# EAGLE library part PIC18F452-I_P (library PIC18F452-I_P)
Microcontroller,PIC18F452-I/P 40MHz Microchip PIC18F452-I/P, 8bit PIC Microcontroller, 40MHz, 32 kB Flash, 40-Pin PDIP Source: Datasheet
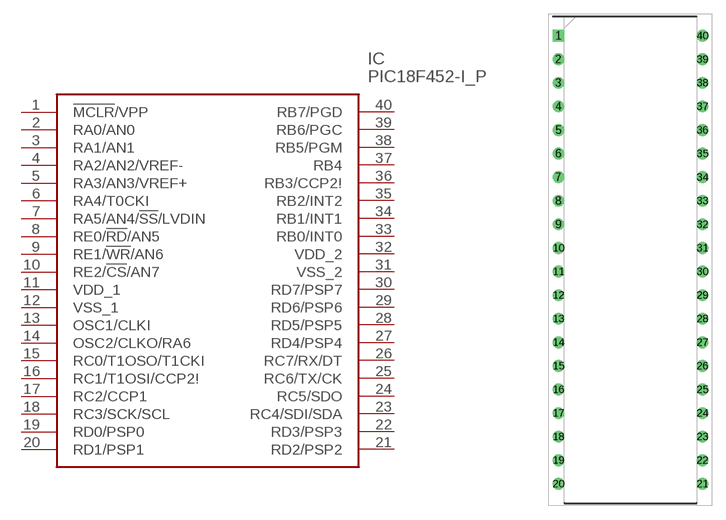
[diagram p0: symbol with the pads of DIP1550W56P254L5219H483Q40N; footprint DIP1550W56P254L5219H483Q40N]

Designator prefix IC

## PIC18F452-I_P (Description: Microcontroller,PIC18F452-I/P 40MHz Microchip PIC18F452-I/P, 8bit PIC Microcontroller, 40MHz, 32 kB Flash, 40-Pin PDIP; Height: 4.83mm; Manufacturer_Name: Microchip; Manufacturer_Part_Number: PIC18F452-I/P; Mouser_Part_Number: 579-PIC18F452-I/P; Mouser_Price-Stock: https://www.mouser.co.uk/ProductDetail/Microchip-Technology-Atmel/PIC18F452-I-P?qs=huzeVNXgovVccIn1hiWGAA%3D%3D)  [DIP1550W56P254L5219H483Q40N]
1  !MCLR!/VPP
2  RA0/AN0
3  RA1/AN1
4  RA2/AN2/VREF-  in
5  RA3/AN3/VREF+  in
6  RA4/T0CKI
7  RA5/AN4/!SS!/LVDIN  in
8  RE0/!RD!/AN5
9  RE1/!WR!/AN6
10  RE2/!CS!/AN7  in
11  VDD_1  pwr
12  VSS_1  pwr
13  OSC1/CLKI  in
14  OSC2/CLKO/RA6  out
15  RC0/T1OSO/T1CKI
16  RC1/T1OSI/CCP2!
17  RC2/CCP1
18  RC3/SCK/SCL
19  RD0/PSP0
20  RD1/PSP1
21  RD2/PSP2
22  RD3/PSP3
23  RC4/SDI/SDA
24  RC5/SDO
25  RC6/TX/CK
26  RC7/RX/DT
27  RD4/PSP4
28  RD5/PSP5
29  RD6/PSP6
30  RD7/PSP7
31  VSS_2  pwr
32  VDD_2  pwr
33  RB0/INT0  in
34  RB1/INT1  in
35  RB2/INT2  in
36  RB3/CCP2!
37  RB4
38  RB5/PGM
39  RB6/PGC
40  RB7/PGD

## Footprint DIP1550W56P254L5219H483Q40N (pad centres in mm)
40-Lead Plastic Dual In-Line (P) - 600 mil Body [PDIP]
drill 0.76 pad 1.16 square: 1 -7.748,24.13
drill 0.76 pad 1.16: 2 -7.748,21.59; 3 -7.748,19.05; 4 -7.748,16.51; 5 -7.748,13.97; 6 -7.748,11.43; 7 -7.748,8.89; 8 -7.748,6.35; 9 -7.748,3.81; 10 -7.748,1.27; 11 -7.748,-1.27; 12 -7.748,-3.81; 13 -7.748,-6.35; 14 -7.748,-8.89; 15 -7.748,-11.43; 16 -7.748,-13.97; 17 -7.748,-16.51; 18 -7.748,-19.05; 19 -7.748,-21.59; 20 -7.748,-24.13; 21 7.748,-24.13; 22 7.748,-21.59; 23 7.748,-19.05; 24 7.748,-16.51; 25 7.748,-13.97; 26 7.748,-11.43; 27 7.748,-8.89; 28 7.748,-6.35; 29 7.748,-3.81; 30 7.748,-1.27; 31 7.748,1.27; 32 7.748,3.81; 33 7.748,6.35; 34 7.748,8.89; 35 7.748,11.43; 36 7.748,13.97; 37 7.748,16.51; 38 7.748,19.05; 39 7.748,21.59; 40 7.748,24.13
